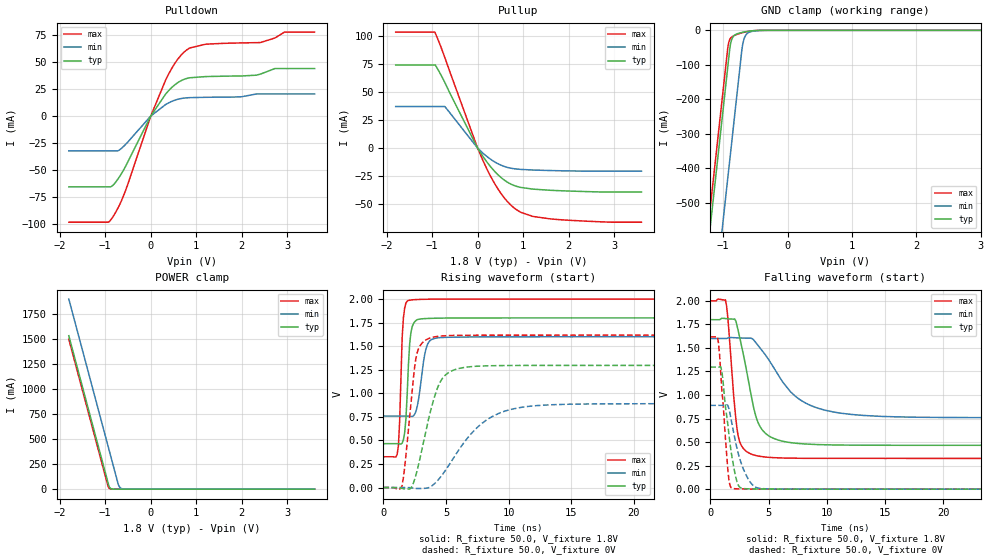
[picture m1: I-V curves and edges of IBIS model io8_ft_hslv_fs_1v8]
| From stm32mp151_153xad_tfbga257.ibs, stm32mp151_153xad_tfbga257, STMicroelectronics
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[Model]   io8_ft_hslv_fs_1v8
Model_type I/O
Polarity   Non-Inverting
Enable   Active-Low
| CAP_THRESHOLD on pad IOFT is "UDTCAPC" :
| Rising=20.00f vddiom   Falling=80.00f vddiom
| C_comp min and max val. don't necessarily correlate with the min and max pvt
| but are the smallest and greatest pad capacitance found.
| var   typ   min   max
C_comp   3.40998pF  3.40231pF  3.47825pF
|C_comp_pullup   1.96225pF  2.05415pF  1.91340pF
|C_comp_pulldown   1.44773pF  1.34816pF  1.56485pF
Vinl = 640.0mV
Vinh = 1.2V
Vmeas = 900.0mV   | Reference voltage for timing measurements
Cref  = 50.0pF   | Timing specification test load capacitance value
Rref  = 100.0MOhm   | Timing specification test load resistance value
Vref  = 0V   | Timing specification test load voltage
[Model Spec]
| TIME_THRESHOLD on pin ZIV11 is "CMOS" :
| Rising=40.00f vdd   Falling=60.00f vdd
Vinl 738.60000mV 665.60000mV 824.60000mV
Vinh 1.04640V 924.40000mV 1.13940V
| variable   typ   min   max
[Temperature Range] 25.0 140.0 -40.0
| variable   typ   min   max
[Voltage Range] 1.8V 1.6V 2.0V
| variable   typ   min   max
[POWER Clamp Reference] 1.8V 1.6V 2.0V
| variable   typ   min   max
[GND Clamp Reference] 0V 0V 0V
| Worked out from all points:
|   slope of the pulldown table from 0 to 0.27 V, typ, clamps not added: 16 ohm
|   slope of the pullup table from 0 to 0.27 V, typ, clamps not added: 17 ohm
|   GND clamp passes 1 mA (typ) near -0.52 V on its own axis
|   POWER clamp passes 1 mA (typ) near -0.83 V on its own axis
|   rising waveform, R_fixture 50.0, V_fixture 1.8V: 20-80 % time 304ps typ, 538ps min, 253ps max; typ from 0.466 V to 1.8 V
|   falling waveform, R_fixture 50.0, V_fixture 1.8V: 20-80 % time 1.36ns typ, 3.3ns min, 669ps max; typ from 1.8 V to 0.466 V
|   rising waveform, R_fixture 50.0, V_fixture 0V: 20-80 % time 1.43ns typ, 3.26ns min, 727ps max; typ from 0 V to 1.3 V
|   falling waveform, R_fixture 50.0, V_fixture 0V: 20-80 % time 802ps typ, 1.13ns min, 566ps max; typ from 1.3 V to 0 V
[POWER Clamp]
-1.8V     1.529A     1.894A     1.494A
-940mV    66.83mA    432.1mA    31.5mA
-910mV    22.88mA    381.1mA    7.077mA
-880mV    7.117mA    330.1mA    1.59mA
-720mV    14.05uA    58.12mA    554nA
-700mV    6.453uA    33.14mA    205nA
-670mV    2.008uA    14.27mA    46.28nA
-610mV    195.3nA    2.645mA    2.496nA
-500mV    3.825nA    120.4uA    129.9pA
3.6V      0A         0A         0A
[GND Clamp]
-1.8V     -1.588A    -1.91A     -1.533A
-1.26V    -670.3mA   -992.4mA   -614.9mA
-1.2V     -568.3mA   -890.4mA   -512.9mA
-930mV    -109.3mA   -431.4mA   -53.86mA
-910mV    -75.33mA   -397.4mA   -32.91mA
-880mV    -34.88mA   -346.4mA   -21.56mA
-810mV    -12.56mA   -227.4mA   -13.55mA
-710mV    -6.275mA   -57.63mA   -7.234mA
-690mV    -5.461mA   -35.21mA   -6.234mA
-650mV    -4.039mA   -14.43mA   -4.463mA
-570mV    -1.908mA   -3.832mA   -1.869mA
3.6V      5.036nA    1.588uA    245.5pA
| variable   typ   min   max
[Pullup Reference] 1.8V 1.6V 2.0V
| variable   typ   min   max
[Pulldown Reference] 0V 0V 0V
[Pullup]
-1.8V     74.35mA    37.17mA    103.8mA
-940mV    74.35mA    37.17mA    103.8mA
-720mV    58.66mA    37.17mA    80.94mA
0V        7.41pA     1.331nA    4.294pA
120mV     -7.602mA   -4.636mA   -11.35mA
300mV     -17.37mA   -10.37mA   -26.31mA
470mV     -24.69mA   -14.42mA   -37.96mA
650mV     -30.35mA   -17.2mA    -47.56mA
820mV     -33.69mA   -18.53mA   -54.05mA
1.21V     -36.65mA   -19.59mA   -61.09mA
1.6V      -37.71mA   -20.06mA   -63.31mA
3.6V      -39.21mA   -20.61mA   -66.25mA
[Pulldown]
-1.8V     -65.8mA    -32.31mA   -98.64mA
-930mV    -65.8mA    -32.31mA   -98.64mA
-850mV    -65.04mA   -32.31mA   -94.81mA
-580mV    -48.83mA   -27.49mA   -72.14mA
0V        0A         -2pA       0A
330mV     20.59mA    10.79mA    33.74mA
560mV     30.02mA    15.15mA    50.81mA
780mV     34.81mA    16.9mA     61.1mA
1.21V     36.69mA    17.44mA    66.81mA
2.41V     38.98mA    20.52mA    68.31mA
2.94V     44.17mA    20.52mA    78.04mA
3.6V      44.17mA    20.52mA    78.04mA
[Ramp]
dV/dt_r 777.74324mV/1.42886ns 533.902mV/3.25464ns 970.01148mV/724.70272ps
dV/dt_f 800.59855mV/1.35908ns 504.72005mV/3.3015ns 1.00395V/666.47973ps
R_load = 50.0
| Removed startup time: 0s 0s 0s  .
| Removed end time: 24.9ns.
[Rising Waveform]
R_fixture   = 50.0
V_fixture   = 1.8V
V_fixture_min = 1.6V
V_fixture_max = 2.0V
0s        465.7mV    758.8mV    326.7mV
1.1ns     465.7mV    758.9mV    353.2mV
1.3ns     463.4mV    759mV      712mV
1.6ns     506.9mV    759.1mV    1.802V
1.9ns     990.8mV    758.8mV    1.979V
2.2ns     1.647V     754.8mV    1.99V
2.8ns     1.785V     928.4mV    1.996V
3.4ns     1.793V     1.47V      1.998V
4.1ns     1.797V     1.583V     1.999V
24.9ns    1.8V       1.6V       2V
| Removed startup time: 0s 0s 0s  .
| Removed end time: 49.9ns.
[Falling Waveform]
R_fixture   = 50.0
V_fixture   = 1.8V
V_fixture_min = 1.6V
V_fixture_max = 2.0V
0s        1.8V       1.6V       2V
1.3ns     1.811V     1.599V     2.01V
1.5ns     1.809V     1.605V     1.829V
2.1ns     1.807V     1.608V     866.6mV
2.4ns     1.681V     1.606V     561.3mV
3.8ns     824.6mV    1.574V     360.8mV
4.9ns     576.1mV    1.396V     339.1mV
7.3ns     488mV      987mV      328.2mV
11.2ns    468.3mV    806.6mV    326.8mV
49.9ns    465.7mV    758.8mV    326.8mV
| Removed startup time: 0s 0s 0s  .
| Removed end time: 49.9ns.
[Rising Waveform]
R_fixture   = 50.0
V_fixture   = 0V
V_fixture_min = 0V
V_fixture_max = 0V
0s        30nV       153nV      -3.193uV
1.5ns     -9.883mV   403.2nV    25.6mV
2.2ns     -6.56mV    -1.689mV   904.2mV
2.6ns     133.3mV    -9.626mV   1.373V
3.9ns     879.2mV    20.27mV    1.593V
4.6ns     1.135V     117.1mV    1.608V
5.5ns     1.24V      293.1mV    1.614V
8ns       1.291V     693.8mV    1.617V
11.2ns    1.296V     854.5mV    1.617V
49.9ns    1.296V     889.8mV    1.617V
| Removed startup time: 0s 0s 0s  .
| Removed end time: 24.9ns.
[Falling Waveform]
R_fixture   = 50.0
V_fixture   = 0V
V_fixture_min = 0V
V_fixture_max = 0V
0s        1.296V     889.9mV    1.617V
700ps     1.296V     889.9mV    1.556V
1ns       1.248V     889.9mV    1.036V
1.5ns     694mV      891.8mV    216.6mV
1.8ns     391.5mV    731.4mV    14.6mV
2.2ns     121.3mV    482.7mV    3.872mV
2.5ns     25.07mV    335.1mV    2.67mV
3.3ns     3.429mV    98.78mV    1.405mV
4.1ns     1.954mV    11.42mV    778.3uV
24.9ns    561.4nV    5.886uV    630.9nV
